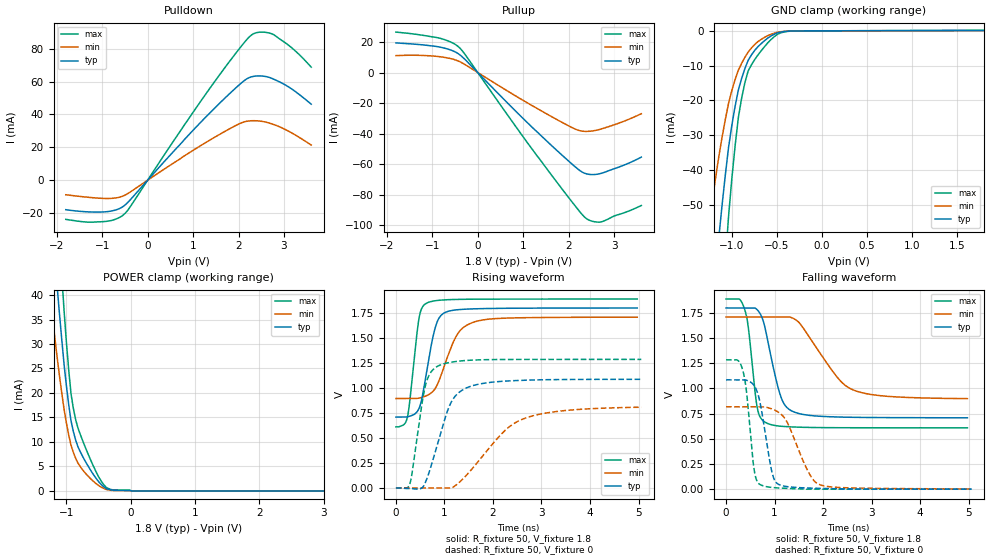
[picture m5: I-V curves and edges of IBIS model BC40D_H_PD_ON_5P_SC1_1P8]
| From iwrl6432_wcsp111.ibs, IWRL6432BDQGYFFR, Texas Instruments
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|   Model Cell BC40D_H_PD_ON_5P_SC1_1P8
|BC40D_H_PD_ON_5P_SC1_1P8
[Model]   BC40D_H_PD_ON_5P_SC1_1P8
Model_type   I/O
Polarity   Non-Inverting
Enable   Active-Low
Vinl =  0.63
Vinh =  1.17
Cref =  15pF
Rref =  100.0000M
Vref =  0V
Vmeas =  0.9
C_comp   2.364487p   2.290698p   2.389419p
|[Input load] weak_pd_on
|[Output drive] slow
|[supplytol] 5
|[temp] ind
[Model Spec]
Vinl   0.63   0.5985   0.6615
Vinh   1.17   1.1115   1.2285
[Temperature Range]   25   125   -40
[Voltage Range]   1.8   1.71   1.89
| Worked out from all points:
|   slope of the pulldown table from 0 to 0.27 V, typ, clamps not added: 32.2 ohm
|   slope of the pullup table from 0 to 0.27 V, typ, clamps not added: 32.6 ohm
|   GND clamp passes 1 mA (typ) near -0.53 V on its own axis
|   POWER clamp passes 1 mA (typ) near -0.43 V on its own axis
|   rising waveform, R_fixture 50, V_fixture 1.8: 20-80 % time 249ps typ, 403ps min, 171ps max; typ from 0.708 V to 1.8 V
|   rising waveform, R_fixture 50, V_fixture 0: 20-80 % time 429ps typ, 920ps min, 246ps max; typ from 0 V to 1.09 V
|   falling waveform, R_fixture 50, V_fixture 1.8: 20-80 % time 310ps typ, 721ps min, 172ps max; typ from 1.8 V to 0.708 V
|   falling waveform, R_fixture 50, V_fixture 0: 20-80 % time 227ps typ, 433ps min, 155ps max; typ from 1.08 V to 0 V
| Nom Voltages:
|   VDD=1.1, VDDS=1.8, VDDS18=1.8, ESD_BIASFET=0, VSS=0, VSSS=0
| Min Voltages:
|   VDD=1.045, VDDS=1.71, VDDS18=1.71, ESD_BIASFET=0, VSS=0, VSSS=0
| Max Voltages:
|   VDD=1.16, VDDS=1.89, VDDS18=1.89, ESD_BIASFET=0, VSS=0, VSSS=0
[POWER_clamp]
|   voltage   I(typ)   I(min)   I(max)
-1.8V     158.9mA    112.5mA    219.9mA
-1.255V   60.04mA    40.04mA    85.04mA
-1.145V   41.99mA    27.45mA    59.9mA
-1.109V   36.4mA     23.66mA    51.97mA
-1.073V   31.03mA    20.08mA    44.3mA
-1.036V   25.91mA    16.71mA    36.9mA
-927.3mV  14.27mA    9.301mA    19.77mA
-854.5mV  10.33mA    6.623mA    14.48mA
-454.5mV  1.273mA    746.6uA    1.931mA
-309.1mV  221.6uA    137.5uA    298.5uA
18.18mV   0A         0A         0A
3.6V      0A         0A         0A
[Pulldown]
|   voltage   I(typ)   I(min)   I(max)
-1.8V     -17.92mA   -8.85mA    -23.8mA
-1.309V   -19.26mA   -10.37mA   -25.5mA
-927.3mV  -19.22mA   -11.12mA   -25.08mA
-654.5mV  -17.65mA   -10.56mA   -23.13mA
-490.9mV  -14.97mA   -8.985mA   -20.05mA
1.364V    40.78mA    24.32mA    55.69mA
2.073V    59.4mA     35mA       81.9mA
2.291V    62.96mA    36.2mA     88.48mA
2.509V    63.41mA    35.84mA    90.12mA
2.782V    61.38mA    33.82mA    88.42mA
3.218V    54.59mA    28.02mA    79.45mA
3.6V      46.26mA    21.39mA    68.79mA
[Pullup]
|   voltage   I(typ)   I(min)   I(max)
-1.8V     19.42mA    11.07mA    26.5mA
-818.2mV  16.58mA    10.3mA     22.34mA
-545.5mV  14.19mA    8.748mA    19.29mA
-381.8mV  11.34mA    6.915mA    15.7mA
1.255V    -37.51mA   -22.64mA   -52.53mA
2.127V    -61.34mA   -36.82mA   -86.78mA
2.291V    -65.12mA   -38.38mA   -92.82mA
2.4V      -66.46mA   -38.59mA   -95.91mA
2.564V    -66.86mA   -38.08mA   -97.75mA
2.727V    -65.99mA   -36.9mA    -97.78mA
3.273V    -60.01mA   -31.26mA   -91.34mA
3.6V      -55.4mA    -26.98mA   -87.12mA
[GND_clamp]
|   voltage   I(typ)   I(min)   I(max)
-1.8V     -270.2mA   -170.2mA   -430.1mA
-1.255V   -91.66mA   -55.91mA   -148.4mA
-1.145V   -59.91mA   -36.45mA   -97.1mA
-1.109V   -50.48mA   -30.83mA   -81.56mA
-1.073V   -41.73mA   -25.65mA   -67.06mA
-1.036V   -33.67mA   -20.93mA   -53.6mA
-927.3mV  -17.08mA   -11.35mA   -25.06mA
-854.5mV  -10.88mA   -7.624mA   -14.94mA
-781.8mV  -6.944mA   -4.956mA   -9.81mA
-636.4mV  -2.852mA   -1.883mA   -4.567mA
-381.8mV  -107.5uA   -92.09uA   -158.2uA
1.8V      101.9uA    59.12uA    150.8uA
[Ramp]
| variable   typ   min   max
dV/dt_f 0.66084962/0.31253884n 0.49607947/0.73684971n 0.77244916/0.17397987n
dV/dt_r 0.65873426/0.43267046n 0.50273236/0.96280761n 0.77696261/0.24769483n
R_load = 50
[Rising Waveform]
R_fixture = 50
V_fixture = 1.8
V_fixture_min = 1.71
V_fixture_max = 1.89
|   time   V(typ)   V(min)   V(max)
0s        708.4mV    893.6mV    610.5mV
233.9ps   710.3mV    893.6mV    701.7mV
279.9ps   716.5mV    893.6mV    844mV
476.5ps   794.9mV    898mV      1.696V
636ps     1.172V     923.1mV    1.847V
782.8ps   1.551V     976.1mV    1.869V
904.7ps   1.709V     1.092V     1.876V
1.252ns   1.78V      1.524V     1.884V
1.574ns   1.789V     1.652V     1.886V
4.974ns   1.798V     1.707V     1.887V
[Rising Waveform]
R_fixture = 50
V_fixture = 0
V_fixture_min = 0
V_fixture_max = 0
|   time   V(typ)   V(min)   V(max)
0s        0V         0V         0V
285.3ps   -5.092mV   0V         39.78mV
603.6ps   50.34mV    0V         1.015V
707ps     191.5mV    0V         1.147V
866.2ps   456.2mV    0V         1.218V
1.158ns   873.3mV    2.78mV     1.258V
1.557ns   1.019V     183.4mV    1.277V
2.249ns   1.068V     574.9mV    1.284V
2.655ns   1.076V     695.6mV    1.284V
5.059ns   1.086V     806.6mV    1.285V
[Falling Waveform]
R_fixture = 50
V_fixture = 1.8
V_fixture_min = 1.71
V_fixture_max = 1.89
|   time   V(typ)   V(min)   V(max)
0s        1.799V     1.708V     1.887V
274.7ps   1.799V     1.708V     1.887V
381.6ps   1.799V     1.708V     1.788V
463.3ps   1.799V     1.708V     1.59V
642.1ps   1.781V     1.708V     811mV
828ps     1.548V     1.708V     658.6mV
1.128ns   919.2mV    1.708V     624.5mV
1.385ns   769.5mV    1.695V     617.1mV
2.586ns   713.3mV    992.4mV    609.5mV
4.974ns   708.1mV    898.7mV    609.1mV
[Falling Waveform]
R_fixture = 50
V_fixture = 0
V_fixture_min = 0
V_fixture_max = 0
|   time   V(typ)   V(min)   V(max)
0s        1.085V     817.5mV    1.284V
345.1ps   1.085V     817.5mV    1.18V
421.6ps   1.081V     817.5mV    967.3mV
578.5ps   1.028V     817.5mV    194mV
705.9ps   847.2mV    817.5mV    44.53mV
942.9ps   174.6mV    796.9mV    17.08mV
1.105ns   42.52mV    755.2mV    11.12mV
1.722ns   10.63mV    148.2mV    0V
1.93ns    7.983mV    44.63mV    0V
5.059ns   0V         2.09mV     0V
